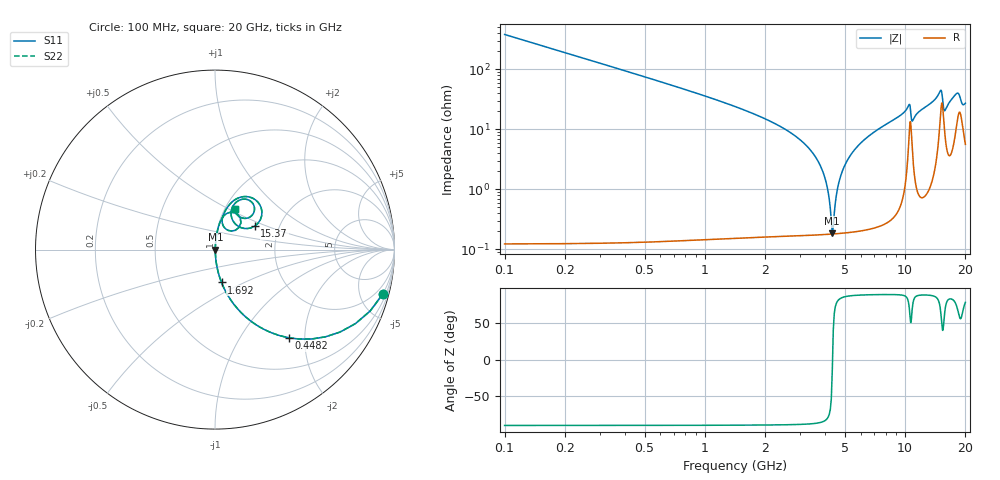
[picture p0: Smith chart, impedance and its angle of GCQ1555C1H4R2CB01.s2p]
!Murata Part Number: GCQ1555C1H4R2CB01
!These Parameters are Measured in Series Mode Connection
!Data Generated on Jan 08, 2026
!  o--ll--o
!Port1  Port2
!  o------o
!Operation Temp=25[degC], DC Bias Voltage=0[V]
!Freq. Start=100[MHz] Stop=20[GHz] 401[Steps]
# Hz S RI R 50
!Freq.(Hz) S11(Real) S11(Imag) S21(Real) S21(Imag) S12(Real) S12(Imag) S22(Real) S22(Imag)
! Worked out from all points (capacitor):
!   401 points, 100 MHz to 20 GHz, reference 50 ohm
!   read as one part in series: C = 4.2 pF near 199.5 MHz
!   lowest |Z| = 187 mohm at 4.329 GHz (marker M1)
!   series resonance near 4.341 GHz, so ESL is about 320 pH
!   S11 on the Smith chart (normalised r, x): 100 MHz: 1.00, -7.57; 448.2 MHz: 1.00, -1.67; 1.692 GHz: 1.00, -0.38; 15.37 GHz: 1.50, +0.42; 20 GHz: 1.11, +0.53
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1e8  0.9348 -0.2468  0.0652 0.2468  0.0652 0.2468  0.9348 -0.2468
4.4825e8  0.4117 -0.4914  0.5883 0.4914  0.5883 0.4914  0.4117 -0.4914
8.96e8  0.1417 -0.347  0.8583 0.347  0.8583 0.347  0.1417 -0.347
1.692e9  0.0363 -0.1829  0.9637 0.1829  0.9637 0.1829  0.0363 -0.1829
3.43325e9  0.00344 -0.0414  0.9966 0.0414  0.9966 0.0414  0.00344 -0.0414
3.9805e9  0.002 -0.0152  0.998 0.0152  0.998 0.0152  0.002 -0.0152
4.32875e9  0.00181 -0.000476  0.9982 0.000476  0.9982 0.000476  0.00181 -0.000476
4.42825e9  0.00183 0.00352  0.9982 -0.00352  0.9982 -0.00352  0.00183 0.00352
4.677e9  0.00201 0.0132  0.998 -0.0132  0.998 -0.0132  0.00201 0.0132
5.02525e9  0.00256 0.0259  0.9974 -0.0259  0.9974 -0.0259  0.00256 0.0259
5.72175e9  0.00445 0.0496  0.9955 -0.0496  0.9955 -0.0496  0.00445 0.0496
6.7665e9  0.00896 0.0819  0.991 -0.0819  0.991 -0.0819  0.00896 0.0819
1.005e10  0.0514 0.1906  0.9486 -0.1906  0.9486 -0.1906  0.0514 0.1906
1.049775e10  0.1271 0.1946  0.8729 -0.1946  0.8729 -0.1946  0.1271 0.1946
1.0846e10  0.0618 0.1136  0.9382 -0.1136  0.9382 -0.1136  0.0618 0.1136
1.338325e10  0.0767 0.2458  0.9233 -0.2458  0.9233 -0.2458  0.0767 0.2458
1.497525e10  0.2271 0.2758  0.7729 -0.2758  0.7729 -0.2758  0.2271 0.2758
1.537325e10  0.2216 0.1311  0.7784 -0.1311  0.7784 -0.1311  0.2216 0.1311
1.57215e10  0.1133 0.1428  0.8867 -0.1428  0.8867 -0.1428  0.1133 0.1428
1.67165e10  0.1033 0.2473  0.8967 -0.2473  0.8967 -0.2473  0.1033 0.2473
1.85075e10  0.2201 0.2279  0.7799 -0.2279  0.7799 -0.2279  0.2201 0.2279
2e10  0.1097 0.2242  0.8903 -0.2242  0.8903 -0.2242  0.1097 0.2242
